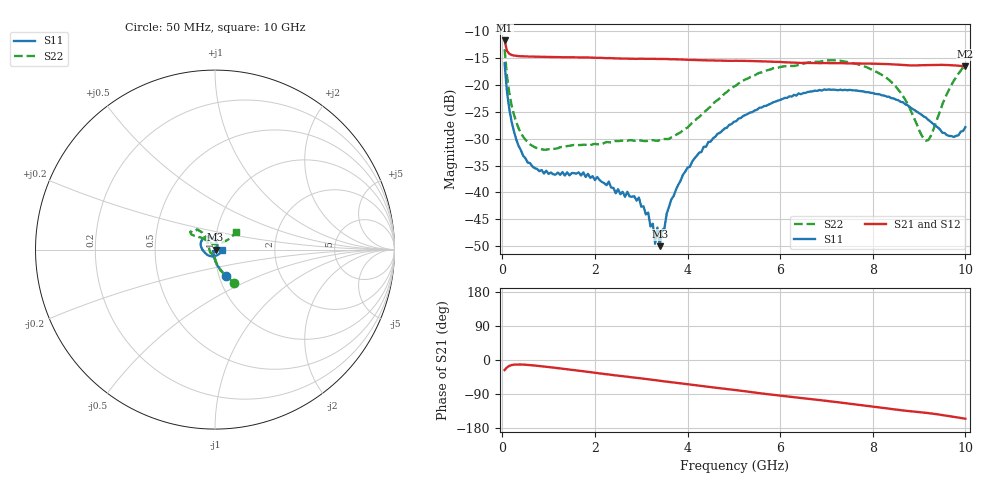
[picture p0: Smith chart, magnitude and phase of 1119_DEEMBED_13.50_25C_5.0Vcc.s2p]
!Hittite Microwave Corp.
!Digital Attenuator/PhaseShifter Rev 1.4.0
!Filename: C:\DATA\DATA\1119_DEEMBED_13.50_25C_5.0Vcc.s2p
!VNA ID: Agilent Technologies,N5224A,MY51441122,A.10.45.03
!Device type:
!2 Port Calibration.
!Temp(C): 25
!Lot Number:
!Serial Number:
!Operator:
!Misc:
!Attenuator:  13.500
# GHZ S DB R 50.0
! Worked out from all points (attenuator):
!   200 points, 50 MHz to 10 GHz, reference 50 ohm
!   highest |S21| = -11.72 dB at 50 MHz (marker M1); lowest = -16.5 dB at 10 GHz (marker M2)
!   lowest |S11| = -50.0 dB at 3.4 GHz (marker M3), VSWR 1.01, Z = 50.3 - j0.101 ohm
!   |S11| at or under -10 dB: start of sweep to end of sweep
!   |S22| runs from -32.0 to -13.3 dB; largest |S21 - S12| = 0.00059
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0.05  -15.95 -68.1  -11.72 -26.4  -11.72 -26.5  -13.34 -60.0
0.1  -21.17 -82.5  -13.63 -19.7  -13.63 -19.7  -18.24 -75.0
0.2  -26.80 -95.3  -14.41 -13.5  -14.42 -13.5  -23.75 -86.2
0.55  -34.45 -119.8  -14.71 -12.9  -14.71 -12.9  -30.67 -99.3
0.9  -36.47 -131.4  -14.77 -17.2  -14.78 -17.2  -32.04 -105.5
1.75  -36.27 -137.2  -14.89 -29.7  -14.89 -29.7  -31.12 -115.2
2.95  -40.95 -97.8  -15.12 -47.7  -15.13 -47.7  -30.33 -152.7
3.2  -46.34 -71.3  -15.13 -51.5  -15.15 -51.6  -30.40 -164.8
3.25  -45.82 -52.5  -15.13 -52.4  -15.14 -52.5  -30.27 -166.9
3.3  -49.55 -49.6  -15.15 -53.2  -15.16 -53.3  -30.35 -170.6
3.35  -46.54 -22.1  -15.16 -54.0  -15.17 -54.0  -30.41 -172.9
3.4  -50.00 -18.6  -15.16 -54.7  -15.17 -54.8  -30.26 -175.1
3.65  -41.30 36.5  -15.23 -58.7  -15.23 -58.7  -29.75 171.2
3.9  -36.73 51.2  -15.27 -62.8  -15.28 -62.8  -28.45 157.1
4.45  -30.60 65.3  -15.44 -71.0  -15.45 -71.0  -24.36 134.3
5.05  -26.75 83.4  -15.50 -79.6  -15.52 -79.6  -20.10 126.6
6.7  -21.18 127.2  -15.90 -103.7  -15.91 -103.7  -15.71 139.7
7.65  -21.03 153.3  -16.00 -117.6  -16.01 -117.6  -16.08 147.3
8.35  -22.20 171.3  -16.13 -128.5  -16.14 -128.5  -19.06 141.3
9.15  -26.08 -139.6  -16.31 -139.3  -16.33 -139.3  -30.37 91.0
9.65  -29.49 -65.7  -16.31 -148.1  -16.33 -148.1  -20.81 37.6
10  -27.85 0.8  -16.54 -154.9  -16.54 -154.9  -16.26 39.4
